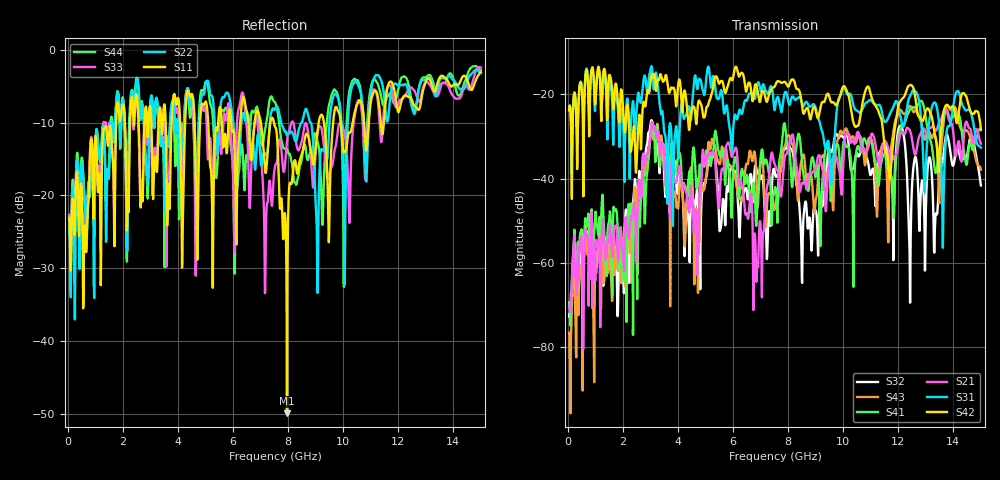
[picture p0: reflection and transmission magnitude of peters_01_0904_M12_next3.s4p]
# MHZ S RI R 50.00
! FREQ  S11  S12  S13  S14
!  S21  S22  S23  S24
!  S31  S32  S33  S34
!  S41  S42  S43  S44
!  REAL  IMAG  REAL  IMAG  REAL  IMAG  REAL  IMAG
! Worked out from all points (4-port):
!   1496 points, 50 MHz to 15 GHz, reference 50 ohm
!   strongest paths, dB at 50 MHz, 3.79 GHz, 7.53 GHz, 11.27 GHz, 15 GHz:
!     S42: -23.8, -18.5, -17.9, -23.8, -28.3
!     S31: -23.8, -36.2, -23.2, -22.5, -32.6
!     S21: -70.6, -35.6, -36.8, -35.7, -31.7
!     S41: -69.4, -31.2, -42.1, -41.4, -28.5
!     S43: -76.7, -40.4, -46.4, -40.6, -37.9
!     S32: -72.3, -32.9, -39.0, -35.0, -41.6
!   lowest |S11| = -50.0 dB at 7.96 GHz (marker M1), VSWR 1.01, Z = 50.1 + j0.293 ohm
!   |S11| at or under -10 dB: start of sweep to 1.758 GHz; 7.487 GHz to 9.112 GHz (1.626 GHz wide, 19.6 % of centre); 9.912 GHz to 10.34 GHz (430.4 MHz wide, 4.25 % of centre)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
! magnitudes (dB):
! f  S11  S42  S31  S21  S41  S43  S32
! 50 MHz  -23.1  -23.8  -23.8  -70.6  -69.4  -76.7  -72.3
! 3.07 GHz  -15.5  -15.1  -14.3  -26.5  -26.5  -28.0  -26.7
! 6.87 GHz  -8.4  -18.5  -18.0  -61.5  -48.4  -43.9  -38.5
! 7.96 GHz  -50.0  -17.7  -20.0  -34.0  -31.6  -29.9  -32.6
! 8.5 GHz  -14.3  -22.4  -21.9  -41.1  -35.6  -35.3  -63.7
! 9.75 GHz  -7.9  -22.6  -25.0  -34.8  -32.0  -32.1  -29.4
! 15 GHz  -3.1  -28.3  -32.6  -31.7  -28.5  -37.9  -41.6
